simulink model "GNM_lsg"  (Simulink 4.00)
settings: Solver=ode45  StartTime=0.0  StopTime=0.2  FixedStep=0.005  RelTol=1e-3
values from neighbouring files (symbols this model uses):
  CE = (2*NA/pi)*2*pi    (= 240)    [GNM_lsg_ini.m]
  CM = 2*NA/pi    (= 38.1971863421)    [GNM_lsg_ini.m]
  Fpwm = 5000    [GNM_lsg_ini.m]
  J = 0.012    [GNM_lsg_ini.m]
  LA = 0.004    [GNM_lsg_ini.m]
  psi = 0.04    [GNM_lsg_ini.m]
  RA = 0.25    [GNM_lsg_ini.m]
  Umax = 200    [GNM_lsg_ini.m]
libraries: simulink3 x1

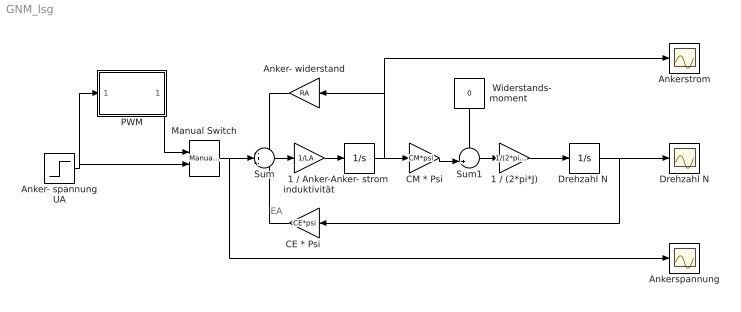
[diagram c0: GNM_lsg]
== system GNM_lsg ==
  note: EA
  " Widerstands-  moment" : Constant  Orientation=down  Value=0
  1 / (2*pi*J) : Gain  Gain=1/(2*pi*J)  Multiplication=Element-wise(K.*u)  SaturateOnIntegerOverflow=on
  1 / Anker- induktivität : Gain  Gain=1/LA  Multiplication=Element-wise(K.*u)  SaturateOnIntegerOverflow=on
  Anker- spannung UA : Step  Time=0.05  Before=0  After=50  SampleTime=0
  Anker- strom : Integrator  ExternalReset=none  InitialConditionSource=internal  InitialCondition=0  LimitOutput=off  UpperSaturationLimit=inf  LowerSaturationLimit=-inf  ShowSaturationPort=off  ShowStatePort=off  AbsoluteTolerance=auto
  Anker- widerstand : Gain  Orientation=left  Gain=RA  Multiplication=Element-wise(K.*u)  SaturateOnIntegerOverflow=on
  Ankerspannung : Scope
  Ankerstrom : Scope
  "CE * Psi " : Gain  Orientation=left  Gain=CE*psi  Multiplication=Element-wise(K.*u)  SaturateOnIntegerOverflow=on
  CM * Psi : Gain  Gain=CM*psi  Multiplication=Element-wise(K.*u)  SaturateOnIntegerOverflow=on
  Drehzahl N : Scope
  "Drehzahl N " : Integrator  ExternalReset=none  InitialConditionSource=internal  InitialCondition=0  LimitOutput=off  UpperSaturationLimit=inf  LowerSaturationLimit=-inf  ShowSaturationPort=off  ShowStatePort=off  AbsoluteTolerance=auto
  Manual Switch : simulink3/Nonlinear/Manual Switch  sw=0  action=0
  PWM : Subsystem
  Sum : Sum  Inputs=-+-  SaturateOnIntegerOverflow=on
  Sum1 : Sum  Inputs=-+|  SaturateOnIntegerOverflow=on
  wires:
  Anker- widerstand/1 -> Sum/1
  Anker- strom/1 -> CM * Psi/1, Anker- widerstand/1, Ankerstrom/1
  Sum/1 -> 1 / Anker- induktivität/1
  1 / Anker- induktivität/1 -> Anker- strom/1
  CM * Psi/1 -> Sum1/2
  Sum1/1 -> 1 / (2*pi*J)/1
  1 / (2*pi*J)/1 -> "Drehzahl N "/1
  " Widerstands-  moment"/1 -> Sum1/1
  "CE * Psi "/1 -> Sum/3
  "Drehzahl N "/1 -> "CE * Psi "/1, Drehzahl N/1
  Manual Switch/1 -> Sum/2, Ankerspannung/1
  PWM/1(UAist) -> Manual Switch/1
  Anker- spannung UA/1 -> PWM/1(UAsoll), Manual Switch/2

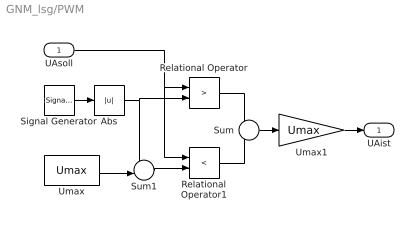
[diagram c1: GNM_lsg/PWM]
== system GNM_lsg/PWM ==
  UAsoll : Inport  Port=1
  Abs : Abs  SaturateOnIntegerOverflow=on
  Relational Operator : RelationalOperator  Operator=>
  Relational Operator1 : RelationalOperator  Operator=<
  Signal Generator : SignalGenerator  WaveForm=sawtooth  Amplitude=Umax  Frequency=Fpwm  Units=Hertz
  Sum : Sum  Inputs=+-  SaturateOnIntegerOverflow=on
  Sum1 : Sum  Inputs=+-|  SaturateOnIntegerOverflow=on
  Umax : Constant  Value=Umax
  Umax1 : Gain  Gain=Umax  Multiplication=Element-wise(K.*u)  SaturateOnIntegerOverflow=on
  UAist : Outport  Port=1  InitialOutput=0
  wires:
  Sum/1 -> Umax1/1
  Umax1/1 -> UAist/1
  Relational Operator1/1 -> Sum/2
  Relational Operator/1 -> Sum/1
  Umax/1 -> Sum1/2
  Abs/1 -> Sum1/1, Relational Operator/2
  UAsoll/1 -> Relational Operator/1, Relational Operator1/1
  Sum1/1 -> Relational Operator1/2
  Signal Generator/1 -> Abs/1
